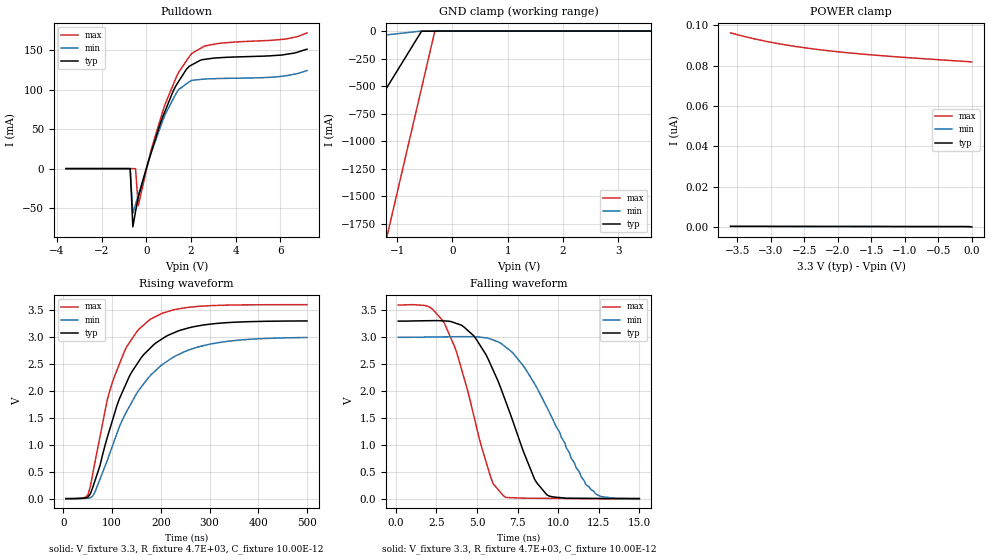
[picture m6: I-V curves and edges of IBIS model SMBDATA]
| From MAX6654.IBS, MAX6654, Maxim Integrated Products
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|   SMBDATA I/O
[Model]   SMBDATA
|Signals   SMBDATA
Model_type   I/O_open_drain
Vinl = 0.80V
Vinh = 2.20V
Polarity   Inverting
Vmeas = 1.65V
C_comp   3.182E-12   2.621E-12   3.676E-12
[Temperature Range]   25   -55   125
[Voltage Range]   3.30V   3.00V   3.60V
[Pullup Reference]   3.30V   3.00V   3.60V
[Pulldown Reference]   0.00V   0.00V   0.00V
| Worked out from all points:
|   slope of the pulldown table from 0 to 0.495 V, typ, clamps not added: 10.9 ohm
|   GND clamp passes 1 mA (typ) near -0.37 V on its own axis
|   rising waveform, V_fixture 3.3, R_fixture 4.7E+03, C_fixture 10.00E-12: 20-80 % time 85.5ns typ, 106ns min, 68.7ns max; typ from 0.007 V to 3.3 V
|   falling waveform, V_fixture 3.3, R_fixture 4.7E+03, C_fixture 10.00E-12: 20-80 % time 2.53ns typ, 3.06ns min, 1.98ns max; typ from 3.3 V to 0.011 V
[Pulldown]
| Note that the [Pulldown] voltage table is referenced to Gnd.
|V(V)   I(typ)   I(min)   I(max)
-3.6V     0A         0A         0A
-720mV    0A         0A         0A
-600mV    -73.76mA   -56.6mA    0A
-480mV    -54.16mA   -45.28mA   0A
-360mV    -36.42mA   -34mA      -47.11mA
240mV     22.27mA    21.6mA     25.88mA
840mV     72.72mA    68.17mA    81.25mA
1.44V     110mA      99.96mA    121.5mA
1.92V     129.5mA    109.8mA    141.6mA
2.64V     138.5mA    113.5mA    155.5mA
5.64V     143.1mA    115.8mA    162.6mA
7.2V      151.3mA    124.2mA    172mA
[POWER_clamp]
| Note that the [POWER_clamp] voltage table is referenced to Vcc
| and is calculated using Vtable=Vcc - Vmeasured.
|V(V)   I(typ)   I(min)   I(max)
-3.6V     375.4pA    373.6pA    96.35nA
-3.44V    369.3pA    367.7pA    94.92nA
-3.28V    363pA      361.6pA    93.64nA
-3V       352.3pA    351.2pA    91.68nA
-2.84V    346.1pA    345.1pA    90.71nA
-2.64V    338.6pA    337.8pA    89.64nA
-2.28V    325pA      324.6pA    88.02nA
-1.84V    308.6pA    308.9pA    86.44nA
-1.4V     292.6pA    293.4pA    85.16nA
-840mV    272.6pA    274.4pA    83.78nA
-40mV     245.6pA    249.1pA    82.04nA
0V        142.7pA    129pA      81.88nA
[GND_clamp]
| Note that the [GND_clamp] voltage table is referenced to Gnd.
|V(V)   I(typ)   I(min)   I(max)
-3.6V     -2.483A    -169.4mA   -7.066A
-2.8V     -1.83A     -124.8mA   -5.343A
-2.72V    -1.765A    -120.3mA   -5.171A
-1.2V     -524.3mA   -35.66mA   -1.897A
-1.12V    -459mA     -31.2mA    -1.725A
-560mV    -1.93mA    -1.784uA   -519.1mA
-320mV    -772.1uA   -713.4nA   -2.201mA
3.6V      372.8pA    463.3pA    81.96nA
[Ramp]
|variable   typ   min   max
dV/dt_r   3.30/8.530E-08   3.00/1.066E-07   3.60/6.877E-08
dV/dt_f   3.30/2.535E-09   3.00/3.064E-09   3.60/1.988E-09
R_load = 4.7E+03
[Rising Waveform]
V_fixture = 3.3
V_fixture_min = 3.0
V_fixture_max = 3.6
R_fixture = 4.7E+03
L_fixture = 0
C_fixture = 10.00E-12
|Time   V(typ)   V(min)   V(max)
5ns       6.94mV     6.134mV    7.46mV
50ns      30.23mV    14.22mV    68.95mV
65ns      346.5mV    136.4mV    698.3mV
90ns      1.141V     714.8mV    1.838V
100ns     1.438V     967.5mV    2.147V
130ns     2.164V     1.625V     2.823V
175ns     2.766V     2.253V     3.304V
225ns     3.072V     2.624V     3.5V
280ns     3.211V     2.824V     3.569V
500ns     3.298V     2.991V     3.599V
[Falling Waveform]
V_fixture = 3.3
V_fixture_min = 3.0
V_fixture_max = 3.6
R_fixture = 4.7E+03
L_fixture = 0
C_fixture = 10.00E-12
|Time   V(typ)   V(min)   V(max)
150ps     3.3V       3V         3.599V
1.95ns    3.308V     3.005V     3.577V
3ns       3.303V     3.009V     3.258V
4.8ns     3.029V     3.012V     1.553V
6ns       2.389V     2.95V      285.6mV
6.75ns    1.828V     2.824V     35.73mV
8.55ns    368.8mV    2.137V     18.43mV
9.3ns     83.23mV    1.707V     16.55mV
11.7ns    15.63mV    273.2mV    13.01mV
15ns      11.48mV    12.94mV    10.55mV
